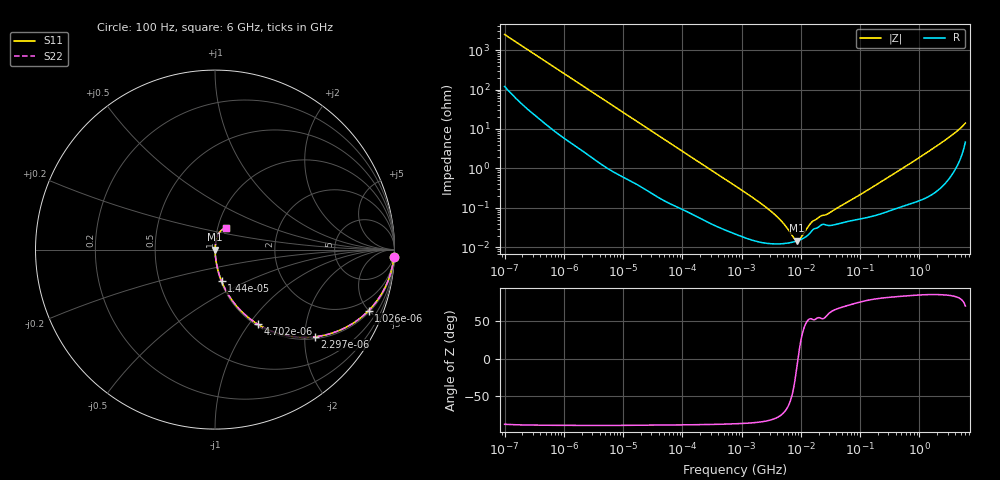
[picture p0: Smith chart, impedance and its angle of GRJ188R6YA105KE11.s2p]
!Murata Part Number: GRJ188R6YA105KE11
!These Parameters are Measured in Series Mode Connection
!Data Generated on Jun 19, 2026
!  o--ll--o
!Port1  Port2
!  o------o
!Operation Temp=25[degC], DC Bias Voltage=0[V]
!Freq. Start=100[Hz] Stop=6[GHz] 401[Steps]
# Hz S RI R 50
!Freq.(Hz) S11(Real) S11(Imag) S21(Real) S21(Imag) S12(Real) S12(Imag) S22(Real) S22(Imag)
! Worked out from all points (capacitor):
!   401 points, 100 Hz to 6 GHz, reference 50 ohm
!   read as one part in series: C = 639 nF near 109 Hz
!   lowest |Z| = 14.8 mohm at 8.692 MHz (marker M1)
!   series resonance near 8.962 MHz, so ESL is about 490 pH
!   S11 on the Smith chart (normalised r, x): 100 Hz: 3, -50; 1.026 kHz: 1.11, -4.98; 2.297 kHz: 1.05, -2.25; 4.702 kHz: 1.02, -1.11; 14.4 kHz: 1.01, -0.37; 6 GHz: 1.09, +0.27
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100  0.9965 -0.04  0.00355 0.04  0.00355 0.04  0.9965 -0.04
350  0.9774 -0.1354  0.0226 0.1354  0.0226 0.1354  0.9774 -0.1354
656  0.9324 -0.2392  0.0676 0.2392  0.0676 0.2392  0.9324 -0.2392
1026  0.8553 -0.3405  0.1447 0.3405  0.1447 0.3405  0.8553 -0.3405
2008  0.6195 -0.4745  0.3805 0.4745  0.3805 0.4745  0.6195 -0.4745
2297  0.5568 -0.4858  0.4432 0.4858  0.4432 0.4858  0.5568 -0.4858
4702  0.2394 -0.4164  0.7606 0.4164  0.7606 0.4164  0.2394 -0.4164
7695  0.109 -0.3009  0.891 0.3009  0.891 0.3009  0.109 -0.3009
14402  0.0366 -0.1758  0.9634 0.1758  0.9634 0.1758  0.0366 -0.1758
40335  0.00619 -0.066  0.9938 0.066  0.9938 0.066  0.00619 -0.066
774597  0.000232 -0.00365  0.9998 0.00365  0.9998 0.00365  0.000232 -0.00365
3394479  0.000124 -0.000735  0.9999 0.000735  0.9999 0.000735  0.000124 -0.000735
5079039  0.000125 -0.000389  0.9999 0.000389  0.9999 0.000389  0.000125 -0.000389
7599586  0.000138 -0.000107  0.9999 0.000107  0.9999 0.000107  0.000138 -0.000107
8692127  0.000146 -1.97e-05  0.9999 1.97e-05  0.9999 1.97e-05  0.000146 -1.97e-05
9941735  0.000158 6.76e-05  0.9998 -6.76e-05  0.9998 -6.76e-05  0.000158 6.76e-05
1.555665e7  0.00027 0.00036  0.9997 -0.00036  0.9997 -0.00036  0.00027 0.00036
2.128304e7  0.000355 0.000501  0.9996 -0.000501  0.9996 -0.000501  0.000355 0.000501
3.045065e7  0.000359 0.000659  0.9996 -0.000659  0.9996 -0.000659  0.000359 0.000659
3.124326e8  0.000875 0.00617  0.9991 -0.00617  0.9991 -0.00617  0.000875 0.00617
2.142435e9  0.00453 0.0401  0.9955 -0.0401  0.9955 -0.0401  0.00453 0.0401
6e9  0.0597 0.1195  0.9403 -0.1195  0.9403 -0.1195  0.0597 0.1195
